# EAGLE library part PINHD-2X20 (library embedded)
PIN HEADER
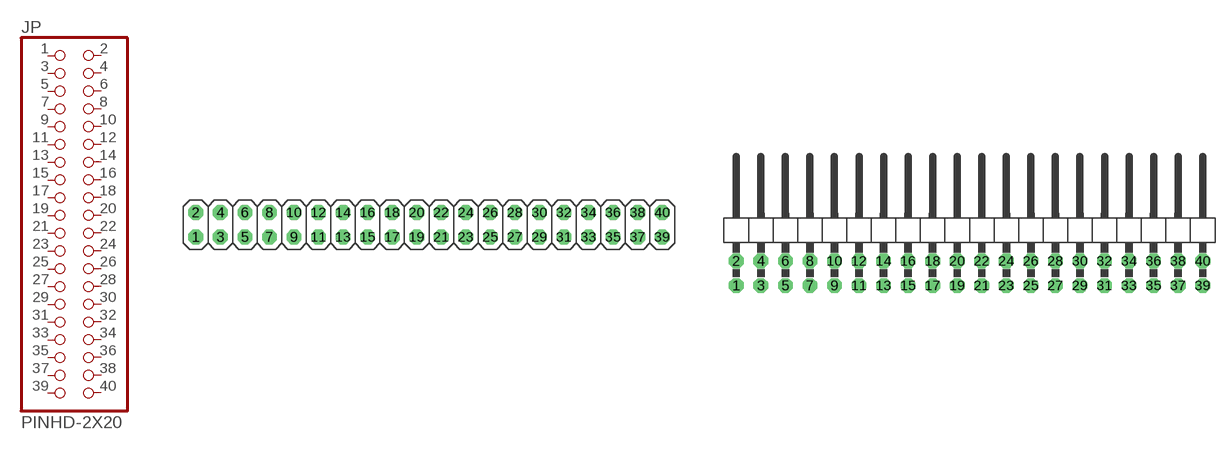
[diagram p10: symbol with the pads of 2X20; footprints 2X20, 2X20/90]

Designator prefix JP

## PINHD-2X20 (ANGLE: Straight; PACKAGE: Pin Header; PITCH: 2.54mm; POS: 40; ROWS: 2)  [2X20]
1  1  pas
2  2  pas
3  3  pas
4  4  pas
5  5  pas
6  6  pas
7  7  pas
8  8  pas
9  9  pas
10  10  pas
11  11  pas
12  12  pas
13  13  pas
14  14  pas
15  15  pas
16  16  pas
17  17  pas
18  18  pas
19  19  pas
20  20  pas
21  21  pas
22  22  pas
23  23  pas
24  24  pas
25  25  pas
26  26  pas
27  27  pas
28  28  pas
29  29  pas
30  30  pas
31  31  pas
32  32  pas
33  33  pas
34  34  pas
35  35  pas
36  36  pas
37  37  pas
38  38  pas
39  39  pas
40  40  pas

## PINHD-2X20/90 (ANGLE: 90; PACKAGE: Pin Header; PITCH: 2.54mm; POS: 40; ROWS: 2)  [2X20/90]
Pads as for 2X20

## Footprint 2X20 (pad centres in mm)
PIN HEADER
drill 1.016 octagon: 1 -24.13,-1.27; 2 -24.13,1.27; 3 -21.59,-1.27; 4 -21.59,1.27; 5 -19.05,-1.27; 6 -19.05,1.27; 7 -16.51,-1.27; 8 -16.51,1.27; 9 -13.97,-1.27; 10 -13.97,1.27; 11 -11.43,-1.27; 12 -11.43,1.27; 13 -8.89,-1.27; 14 -8.89,1.27; 15 -6.35,-1.27; 16 -6.35,1.27; 17 -3.81,-1.27; 18 -3.81,1.27; 19 -1.27,-1.27; 20 -1.27,1.27; 21 1.27,-1.27; 22 1.27,1.27; 23 3.81,-1.27; 24 3.81,1.27; 25 6.35,-1.27; 26 6.35,1.27; 27 8.89,-1.27; 28 8.89,1.27; 29 11.43,-1.27; 30 11.43,1.27; 31 13.97,-1.27; 32 13.97,1.27; 33 16.51,-1.27; 34 16.51,1.27; 35 19.05,-1.27; 36 19.05,1.27; 37 21.59,-1.27; 38 21.59,1.27; 39 24.13,-1.27; 40 24.13,1.27

## Footprint 2X20/90 (pad centres in mm)
PIN HEADER
drill 1.016 octagon: 1 -24.13,-6.35; 2 -24.13,-3.81; 3 -21.59,-6.35; 4 -21.59,-3.81; 5 -19.05,-6.35; 6 -19.05,-3.81; 7 -16.51,-6.35; 8 -16.51,-3.81; 9 -13.97,-6.35; 10 -13.97,-3.81; 11 -11.43,-6.35; 12 -11.43,-3.81; 13 -8.89,-6.35; 14 -8.89,-3.81; 15 -6.35,-6.35; 16 -6.35,-3.81; 17 -3.81,-6.35; 18 -3.81,-3.81; 19 -1.27,-6.35; 20 -1.27,-3.81; 21 1.27,-6.35; 22 1.27,-3.81; 23 3.81,-6.35; 24 3.81,-3.81; 25 6.35,-6.35; 26 6.35,-3.81; 27 8.89,-6.35; 28 8.89,-3.81; 29 11.43,-6.35; 30 11.43,-3.81; 31 13.97,-6.35; 32 13.97,-3.81; 33 16.51,-6.35; 34 16.51,-3.81; 35 19.05,-6.35; 36 19.05,-3.81; 37 21.59,-6.35; 38 21.59,-3.81; 39 24.13,-6.35; 40 24.13,-3.81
